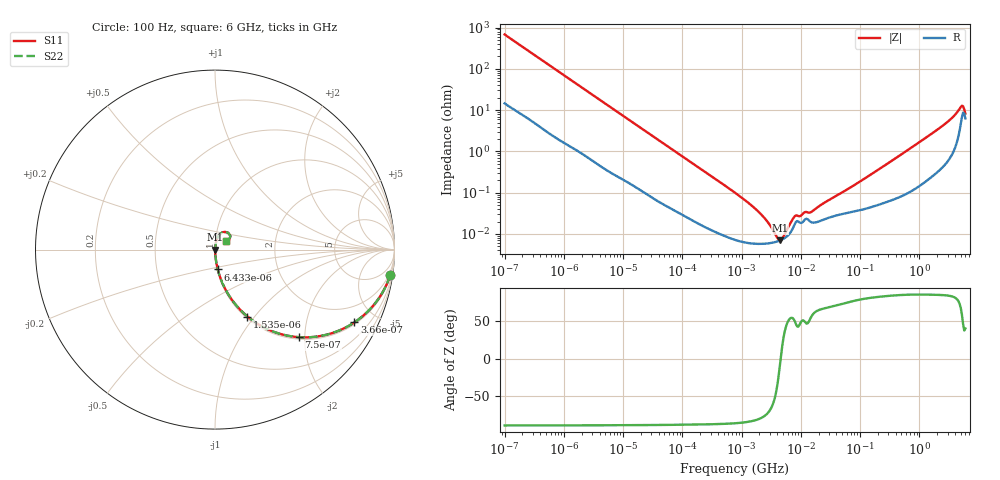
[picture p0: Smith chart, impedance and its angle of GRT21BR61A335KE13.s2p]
!Murata Part Number: GRT21BR61A335KE13
!These Parameters are Measured in Series Mode Connection
!Data Generated on Jun 19, 2026
!  o--ll--o
!Port1  Port2
!  o------o
!Operation Temp=25[degC], DC Bias Voltage=0[V]
!Freq. Start=100[Hz] Stop=6[GHz] 401[Steps]
# Hz S RI R 50
!Freq.(Hz) S11(Real) S11(Imag) S21(Real) S21(Imag) S12(Real) S12(Imag) S22(Real) S22(Imag)
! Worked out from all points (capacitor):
!   401 points, 100 Hz to 6 GHz, reference 50 ohm
!   read as one part in series: C = 2.33 uF near 109 Hz
!   lowest |Z| = 7.05 mohm at 4.441 MHz (marker M1)
!   series resonance near 4.571 MHz, so ESL is about 520 pH
!   S11 on the Smith chart (normalised r, x): 100 Hz: 1, -14; 366 Hz: 1.08, -3.78; 750 Hz: 1.04, -1.87; 1.535 kHz: 1.02, -0.92; 6.433 kHz: 1.01, -0.22; 6 GHz: 1.13, +0.11
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100  0.9759 -0.1429  0.0241 0.1429  0.0241 0.1429  0.9759 -0.1429
205  0.9134 -0.2703  0.0866 0.2703  0.0866 0.2703  0.9134 -0.2703
366  0.7765 -0.4055  0.2235 0.4055  0.2235 0.4055  0.7765 -0.4055
750  0.4661 -0.4878  0.5339 0.4878  0.5339 0.4878  0.4661 -0.4878
1535  0.1808 -0.3728  0.8192 0.3728  0.8192 0.3728  0.1808 -0.3728
2008  0.1172 -0.3093  0.8828 0.3093  0.8828 0.3093  0.1172 -0.3093
6433  0.0153 -0.1103  0.9847 0.1103  0.9847 0.1103  0.0153 -0.1103
40335  0.000941 -0.0185  0.9991 0.0185  0.9991 0.0185  0.000941 -0.0185
774597  7.3e-05 -0.000997  0.9999 0.000997  0.9999 0.000997  7.3e-05 -0.000997
1983483  5.77e-05 -0.000329  0.9999 0.000329  0.9999 0.000329  5.77e-05 -0.000329
2594782  5.85e-05 -0.000211  0.9999 0.000211  0.9999 0.000211  5.85e-05 -0.000211
3712478  6.39e-05 -7.48e-05  0.9999 7.48e-05  0.9999 7.48e-05  6.39e-05 -7.48e-05
4440638  6.97e-05 -1.04e-05  0.9999 1.04e-05  0.9999 1.04e-05  6.97e-05 -1.04e-05
5079039  7.65e-05 3.86e-05  0.9999 -3.86e-05  0.9999 -3.86e-05  7.65e-05 3.86e-05
5554849  8.31e-05 7.25e-05  0.9999 -7.25e-05  0.9999 -7.25e-05  8.31e-05 7.25e-05
7947587  0.000177 0.000206  0.9998 -0.000206  0.9998 -0.000206  0.000177 0.000206
1.555665e7  0.00019 0.000298  0.9998 -0.000298  0.9998 -0.000298  0.00019 0.000298
3.124326e8  0.000656 0.00538  0.9993 -0.00538  0.9993 -0.00538  0.000656 0.00538
2.450438e9  0.00574 0.0408  0.9943 -0.0408  0.9943 -0.0408  0.00574 0.0408
3.505958e9  0.0118 0.0617  0.9882 -0.0617  0.9882 -0.0617  0.0118 0.0617
5.016141e9  0.0546 0.0992  0.9454 -0.0992  0.9454 -0.0992  0.0546 0.0992
6e9  0.0617 0.0469  0.9383 -0.0469  0.9383 -0.0469  0.0617 0.0469
